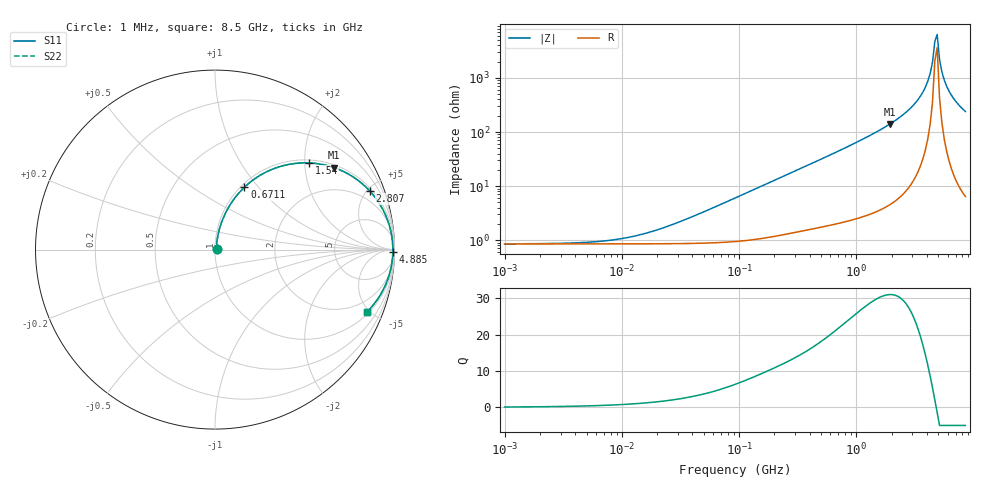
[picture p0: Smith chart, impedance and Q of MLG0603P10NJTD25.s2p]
! S-Parameter Data Generated by TDK Corporation
! Copyright(C) 2025 TDK Corporation.
! All Rights Reserved.
! TDK P/N: MLG0603P10NJTD25 (SMD / SMT Inductor (Coil))
! Property: L=10nH at 500MHz
! Size(LxWxT): 0.6x0.3x0.3mm
! Model Type: s2p (Touchstone File Format Version 1.0)
! Frequency: DC=Yes Start=1MHz Stop=8500MHz 198points Log-sweep
! Model Generated on Feb. 6, 2025
! Terms and conditions regarding TDK Simulation Models:
! 1)This simulation model is being provided solely for informational
!  purposes. Please refer to the specifications of the products in
!  terms of detailed characteristics of such products.
! 2)In no event shall TDK Corporation of any of its subsidiaries be
!  liable for any loss or damage arising, directly or indirectly,
!  from any information contained in this simulation model, including,
!  but not limited to loss or damages arising from any inaccuracies,
!  omissions or errors in connection with such information.
! 3)Any and all copyrights on this simulation model are owned by
!  TDK Corporation.  Duplication or redistribution of this simulation
!  model without prior written permission from TDK Corporation
!  is prohibited.
! 4)This simulation model is subject to any modification or change
!  without any prior notice.
! 5)Neither TDK Corporation nor any of its subsidiaries shall make any
!  warranty, express or implied, including but not limited to the
!  correctness, implied warranties of merchantability and fitness for
!  a particular purpose with respect to this simulation models.
! 6)The use of this simulation model shall be deemed to have consented
!  to the terms and conditions hereof.
! Port Assignments:
!  1 ---@@@--- 2
! Applicable Conditions:
!  Temperature = 25 degC
!  DC Bias Current = 0 A
!  Small Signal Operation
# Hz S MA R 50
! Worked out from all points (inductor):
!   197 points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, 1 MHz to 8.5 GHz, reference 50 ohm
!   read as one part in series: L = 10.3 nH near 42.06 MHz
!   highest Q = 31 at 1.94 GHz (marker M1), where L = 11.6 nH
!   self-resonance near 4.664 GHz
!   S11 on the Smith chart (normalised r, x): 1 MHz: 1.02, +0.00; 671.1 MHz: 1.04, +0.85; 1.54 GHz: 1.07, +2.10; 2.807 GHz: 1.19, +5.19; 4.885 GHz: open; 8.5 GHz: 1.13, -4.80
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1000000  0.008453 4.3  0.9916 -0.0  0.9916 -0.0  0.008453 4.3
4587603  0.008927 19.0  0.9916 -0.2  0.9916 -0.2  0.008927 19.0
1.005548e7  0.01061 36.9  0.9915 -0.4  0.9915 -0.4  0.01061 36.9
2.10461e7  0.01591 57.0  0.9914 -0.8  0.9914 -0.8  0.01591 57.0
9.219544e7  0.05932 77.6  0.989 -3.4  0.989 -3.4  0.05932 77.6
4.229561e8  0.2536 71.9  0.9521 -14.7  0.9521 -14.7  0.2536 71.9
6.710824e8  0.3835 64.8  0.9057 -22.5  0.9057 -22.5  0.3835 64.8
1.016736e9  0.538 55.3  0.8225 -32.5  0.8225 -32.5  0.538 55.3
1.540426e9  0.7123 42.7  0.6786 -45.4  0.6786 -45.4  0.7123 42.7
1.940355e9  0.8045 34.6  0.5687 -53.5  0.5687 -53.5  0.8045 34.6
2.80715e9  0.9219 20.8  0.3552 -67.1  0.3552 -67.1  0.9219 20.8
3.535948e9  0.9679 11.9  0.2059 -75.2  0.2059 -75.2  0.9679 11.9
4.061159e9  0.9839 6.5  0.1132 -78.6  0.1132 -78.6  0.9839 6.5
4.253027e9  0.9872 4.7  0.0821 -78.7  0.0821 -78.7  0.9872 4.7
4.453958e9  0.9895 2.9  0.05103 -76.7  0.05103 -76.7  0.9895 2.9
4.664383e9  0.9908 1.1  0.02083 -63.1  0.02083 -63.1  0.9908 1.1
4.884749e9  0.991 -0.7  0.01553 54.3  0.01553 54.3  0.991 -0.7
5.115526e9  0.9902 -2.5  0.04507 76.2  0.04507 76.2  0.9902 -2.5
5.357206e9  0.9884 -4.3  0.07617 79.1  0.07617 79.1  0.9884 -4.3
5.610304e9  0.9856 -6.1  0.1074 79.2  0.1074 79.2  0.9856 -6.1
6.748056e9  0.9639 -13.4  0.2316 74.4  0.2316 74.4  0.9639 -13.4
8.5e9  0.9144 -22.4  0.3811 66.1  0.3811 66.1  0.9144 -22.4
